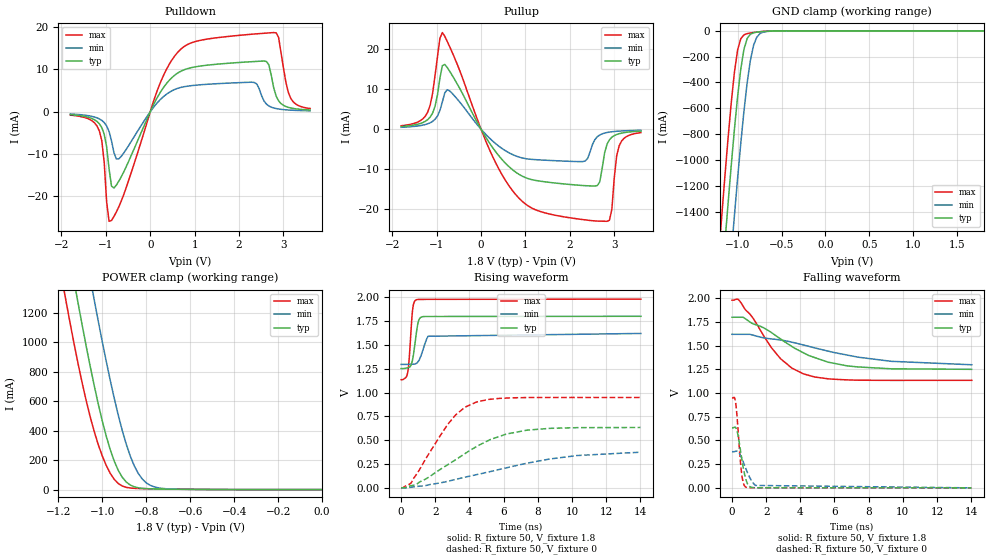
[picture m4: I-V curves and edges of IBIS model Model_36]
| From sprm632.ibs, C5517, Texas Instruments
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| Model based on original model for BC3350CTHYPD
|   Sub model PD_OFF_IND_1P8
[model]   Model_36
|[Description]  [1.8V-I/O-PD_OFF-X, IND]
|   PD_OFF,IND,
|[Input Load]   PD_OFF
|[Output Drive]
|Voltage   1.8V
|Mode   I/O
Model_type   I/O
Polarity   Non-Inverting
Enable   Active-Low
Vinl =  0.63
Vinh =  1.17
Cref =  15.0000pF
Rref =  100.0000M
Vref =  0V
Vmeas =  0.9
C_comp   1.505438p   1.4840531p   1.52103p
[Model Spec]
Vinl   0.63   0.567   0.693
Vinh   1.17   1.053   1.287
[Temperature Range]   25   105   -40
[Voltage Range]   1.8   1.62   1.98
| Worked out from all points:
|   slope of the pulldown table from 0 to 0.27 V, typ, clamps not added: 51 ohm
|   slope of the pullup table from 0 to 0.27 V, typ, clamps not added: 57.1 ohm
|   GND clamp passes 1 mA (typ) near -0.59 V on its own axis
|   POWER clamp passes 1 mA (typ) near -0.52 V on its own axis
|   rising waveform, R_fixture 50, V_fixture 1.8: 20-80 % time 261ps typ, 379ps min, 195ps max; typ from 1.25 V to 1.8 V
|   rising waveform, R_fixture 50, V_fixture 0: 20-80 % time 3.48ns typ, 5.71ns min, 2.09ns max; typ from 0.001 V to 0.634 V
|   falling waveform, R_fixture 50, V_fixture 1.8: 20-80 % time 3.23ns typ, 5.09ns min, 2.09ns max; typ from 1.8 V to 1.25 V
|   falling waveform, R_fixture 50, V_fixture 0: 20-80 % time 357ps typ, 551ps min, 247ps max; typ from 0.634 V to 0 V
[POWER_clamp]
-1.8V     7.656A     8.299A     7.195A
-1.182V   1.868A     2.514A     1.416A
-1.164V   1.711A     2.354A     1.267A
-1.127V   1.405A     2.039A     981.3mA
-1.109V   1.256A     1.883A     846.6mA
-1.036V   703.1mA    1.284A     392.2mA
-963.6mV  270.2mA    740.6mA    110.2mA
-909.1mV  83.65mA    400.5mA    24.3mA
-872.7mV  31.2mA     227.3mA    10.88mA
-836.4mV  12.3mA     109.9mA    7.425mA
-763.6mV  4.548mA    18.58mA    5.183mA
0V        170.6pA    2.308nA    119.6pA
[Pulldown]
-1.8V     -681.9uA   -528.3uA   -794.7uA
-1.145V   -2.848mA   -1.688mA   -4.553mA
-927.3mV  -13.49mA   -4.672mA   -25.91mA
-872.7mV  -17.57mA   -6.855mA   -25.72mA
-709.1mV  -16.44mA   -11.17mA   -22.51mA
218.2mV   4.45mA     2.794mA    6.638mA
818.2mV   10.13mA    6.022mA    15.79mA
2.345V    11.88mA    6.92mA     18.39mA
2.618V    11.89mA    1.797mA    18.61mA
2.836V    3.687mA    752.6uA    18.66mA
3.164V    900.6uA    382.8uA    3.183mA
3.6V      416.6uA    227.7uA    766.1uA
[Pullup]
-1.8V     683.6uA    489.2uA    876.7uA
-1.2V     2.423mA    1.368mA    4.325mA
-1.036V   5.753mA    2.495mA    13.46mA
-872.7mV  15.87mA    6.82mA     24.17mA
-709.1mV  14.53mA    9.611mA    20.69mA
327.3mV   -5.597mA   -3.586mA   -8.356mA
1.145V    -12.6mA    -7.535mA   -19.72mA
2.345V    -14.1mA    -7.933mA   -22.66mA
2.618V    -14.07mA   -1.864mA   -22.95mA
2.891V    -2.623mA   -708.3uA   -22.76mA
3.109V    -1.114mA   -461.7uA   -4.16mA
3.6V      -465.4uA   -255.6uA   -836.2uA
[GND_clamp]
-1.8V     -7.797A    -8.487A    -7.298A
-1.218V   -2.296A    -3.009A    -1.771A
-1.182V   -1.972A    -2.683A    -1.449A
-1.145V   -1.654A    -2.361A    -1.137A
-1.109V   -1.345A    -2.044A    -838.3mA
-1.036V   -766.6mA   -1.434A    -323.5mA
-1V       -511.1mA   -1.144A    -149.1mA
-927.3mV  -142.6mA   -620.4mA   -31.17mA
-854.5mV  -26.4mA    -229.1mA   -16.81mA
-818.2mV  -14.96mA   -112.4mA   -13.02mA
-709.1mV  -5.146mA   -10.44mA   -4.53mA
1.8V      170.6pA    3.271uA    70.6pA
[Ramp]
dV/dt_f 0.33494287/3.2873899n 0.19908904/5.3399226n 0.51436147/2.1136182n
dV/dt_r   0.380584/3.482913n  0.22884863/5.8863639n 0.56965454/2.0907151n
R_load = 50
[Rising Waveform]
R_fixture = 50
V_fixture = 1.8
V_fixture_min = 1.62
V_fixture_max = 1.98
0s        1.252V     1.295V     1.135V
298ps     1.257V     1.296V     1.162V
387.5ps   1.26V      1.296V     1.213V
477ps     1.265V     1.297V     1.369V
662ps     1.339V     1.297V     1.854V
753.1ps   1.439V     1.298V     1.944V
894.7ps   1.63V      1.307V     1.974V
1.092ns   1.78V      1.356V     1.977V
1.575ns   1.798V     1.59V      1.978V
14.03ns   1.8V       1.62V      1.98V
[Rising Waveform]
R_fixture = 50
V_fixture = 0
V_fixture_min = 0
V_fixture_max = 0
0s        659.3uV    355uV      947.1uV
588.7ps   22.95mV    7.206mV    53.82mV
2.425ns   209.8mV    57.22mV    586.1mV
3.194ns   296.2mV    89.17mV    766.6mV
3.742ns   360.2mV    112.4mV    847mV
4.42ns    435.2mV    139.3mV    901.5mV
6.162ns   564.9mV    210.6mV    942.4mV
7.359ns   605.5mV    258.7mV    947.5mV
10.3ns    631.9mV    339.5mV    948.6mV
14.01ns   633.6mV    373.8mV    948.3mV
[Falling Waveform]
R_fixture = 50
V_fixture = 1.8
V_fixture_min = 1.62
V_fixture_max = 1.98
0s        1.8V       1.62V      1.98V
434.9ps   1.8V       1.62V      1.975V
1.214ns   1.733V     1.612V     1.795V
1.877ns   1.686V     1.582V     1.599V
2.839ns   1.571V     1.56V      1.363V
4.179ns   1.425V     1.508V     1.203V
5.63ns    1.326V     1.442V     1.15V
6.761ns   1.286V     1.4V       1.139V
9.317ns   1.256V     1.335V     1.134V
14.03ns   1.251V     1.299V     1.134V
[Falling Waveform]
R_fixture = 50
V_fixture = 0
V_fixture_min = 0
V_fixture_max = 0
0s        633.9mV    381.3mV    949mV
191.7ps   639.7mV    385.1mV    924.4mV
325ps     580.8mV    384.4mV    685.6mV
475.2ps   421.1mV    350mV      316.7mV
556.8ps   324.7mV    319.7mV    163.3mV
658.2ps   214.1mV    274.6mV    55mV
838.5ps   74.01mV    189.5mV    5.783mV
989.7ps   20.11mV    127.1mV    1.898mV
1.377ns   1.033mV    25.51mV    1.324mV
14.01ns   0V         15.16uV    0V
